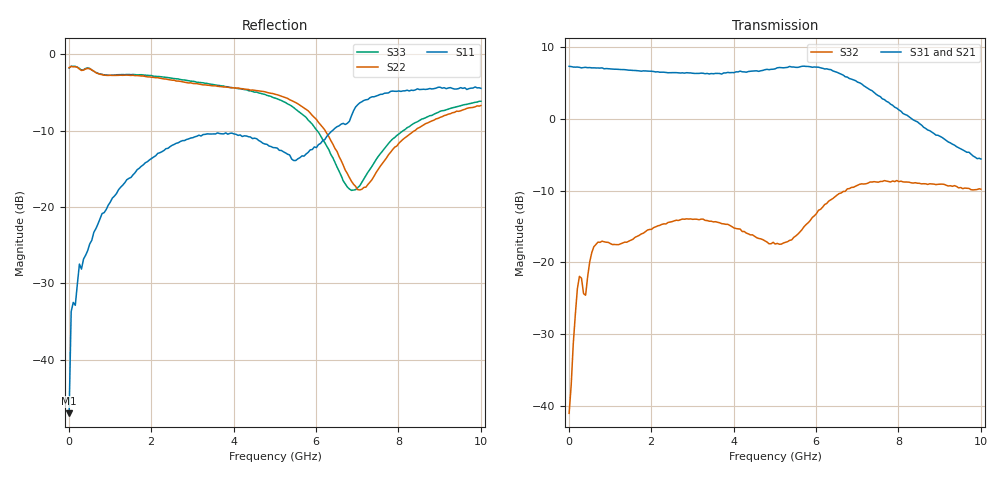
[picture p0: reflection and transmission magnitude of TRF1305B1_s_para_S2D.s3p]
! Created Thu Apr 18 17:47:57 2024
# hz S ri R 50
! 3 Port Network Data from SP1.SP block
!port 1 - INP, port 2 - OUTM, port3 - OUTP
! freq  reS11  imS11  reS12  imS12  reS13  imS13
!  reS21  imS21
!  reS22  imS22  reS23  imS23
!  reS31  imS31  reS32  imS32
!  reS33  imS33
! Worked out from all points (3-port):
!   201 points, 10 MHz to 10 GHz, reference 50 ohm
!   strongest paths, dB at 10 MHz, 2.51 GHz, 5.01 GHz, 7.51 GHz, 10 GHz:
!     S31: 7.3, 6.4, 7.0, 3.2, -5.6
!     S21: 7.4, 6.1, 6.8, 3.1, -5.7
!     S32: -41.0, -14.3, -17.4, -8.8, -9.8
!   lowest |S11| = -47.0 dB at 10 MHz (marker M1), VSWR 1.01, Z = 50.2 + j0.377 ohm
!   |S11| at or under -10 dB: start of sweep to 6.398 GHz
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1e7  0.00241 0.00375  -0.00115 0.015  -0.0014 -0.00468
     -2.331 0.00151  -0.8182 -0.00747  -0.0143 0.0121
     2.32 0.00647  -0.00732 0.00503  -0.8123 0.00998
6e7  -0.0193 -0.00742  0.00445 0.00377  -0.0037 -0.00277
     -2.32 0.1016  -0.8313 0.0341  -0.0117 0.0144
     2.308 -0.1037  -0.00709 0.012  -0.8353 0.0253
6.1e8  -0.0315 -0.0606  0.016 0.0285  0.00946 0.0218
       -2.097 0.9022  -0.7371 0.2402  0.0724 0.101
       2.107 -0.8286  0.0776 0.1023  -0.7396 0.2283
2.56e9  -0.2115 -0.1461  0.0744 0.0101  0.0491 -0.00781
        0.00236 2.013  -0.3975 0.5464  0.1956 -0.00279
        0.1344 -2.093  0.1946 -0.00445  -0.4348 0.5398
3.86e9  -0.2967 -0.0423  0.0812 -0.0333  0.032 -0.0523
        1.292 1.544  -0.1342 0.5928  0.1154 -0.1338
        -1.289 -1.665  0.1215 -0.1384  -0.1564 0.592
5.01e9  -0.2441 0.0136  0.0732 -0.064  -0.0194 -0.059
        2.157 0.3532  0.1146 0.5347  -0.0711 -0.0901
        -2.189 -0.4157  -0.0769 -0.1099  0.0907 0.5082
5.76e9  -0.2145 -0.0595  0.0616 -0.0928  -0.0455 -0.0313
        2.09 -0.9108  0.2402 0.3633  -0.1392 0.081
        -2.14 0.887  -0.1697 0.0699  0.1856 0.3388
6.66e9  -0.326 -0.1348  0.0166 -0.1222  -0.0334 0.00745
        0.7107 -1.867  0.1321 0.1339  0.0241 0.2838
        -0.7179 1.883  -0.000642 0.312  0.0666 0.1326
7.81e9  -0.5718 0.00154  -0.0464 -0.0972  -0.00881 0.0139
        -0.5916 -1.108  -0.0755 0.2155  0.277 0.1912
        0.6337 1.094  0.2884 0.2204  -0.1305 0.2368
1e10  -0.5118 0.3099  -0.0677 -0.0299  -0.000932 0.00928
      -0.5108 -0.0719  0.0637 0.4575  0.2915 -0.059
      0.5243 0.0245  0.3194 -0.0496  0.018 0.4924
